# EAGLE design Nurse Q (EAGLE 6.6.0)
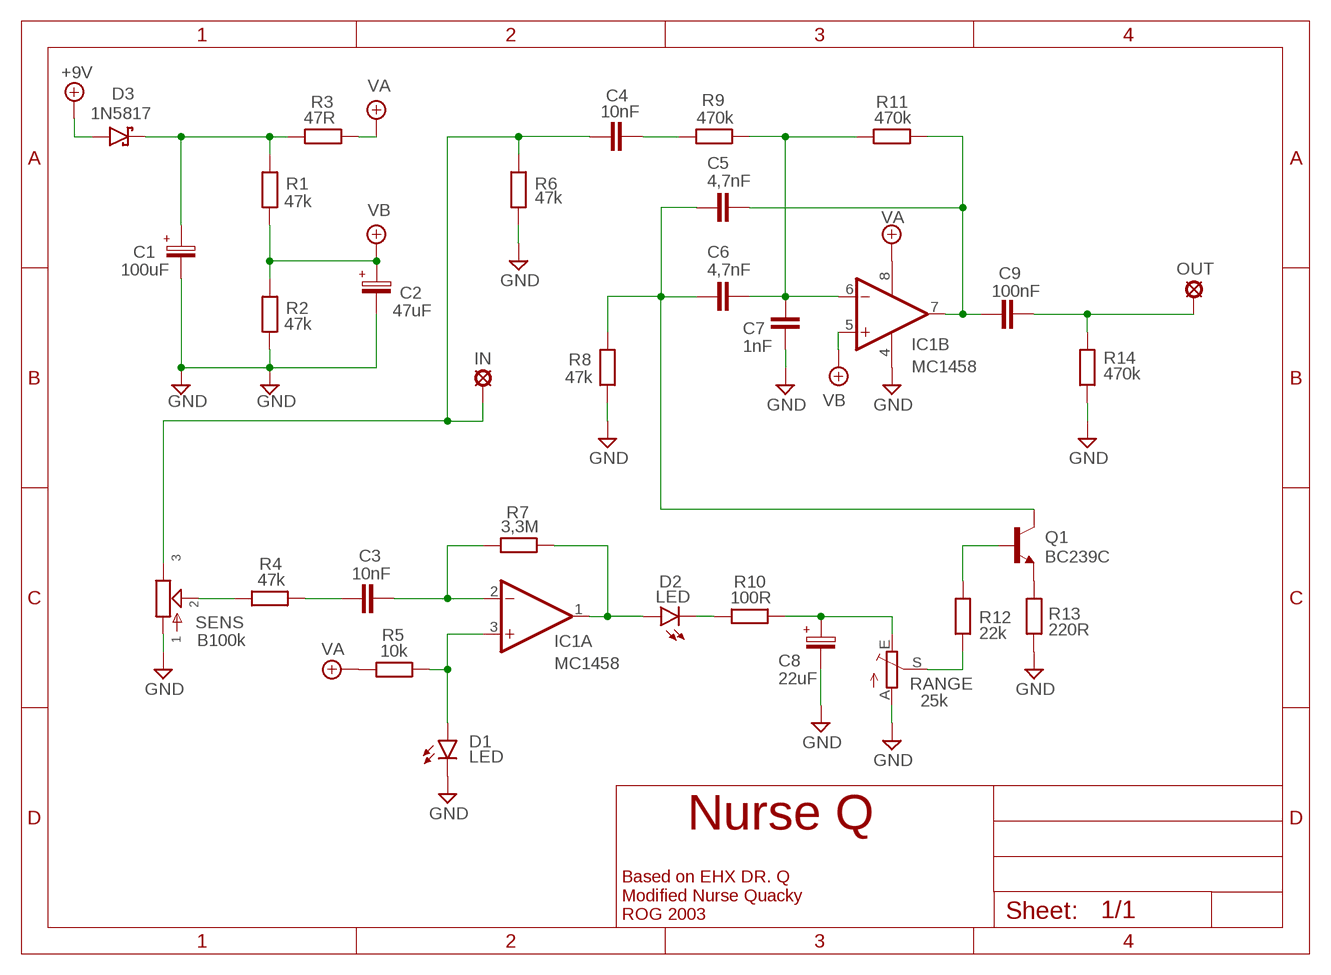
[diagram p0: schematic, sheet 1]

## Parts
+9V  +9V  +9V(T)1  [ROUND]
C1  100uF  063-EU  [063_025]
C2  47uF  063-EU  [063_025]
C3  10nF  1NF-15NF  [3,5MM]
C4  10nF  1NF-15NF  [3,5MM]
C5  4,7nF  1NF-15NF  [3,5MM]
C6  4,7nF  1NF-15NF  [3,5MM]
C7  1nF  1NF-15NF  [3,5MM]
C8  22uF  063-EU  [063_025]
C9  100nF  100NF-220NF  [7,5MM]
D1  LED  LED3MM  [LED3MM]
D2  LED  LED3MM  [LED3MM]
D3  1N5817  [DO41-3]
GND  GND  GND(T)1  [ROUND]
GND1  GND  GND(T)1  [ROUND]
IC1  MC1458  TL072P  [DIL08]
IN  MCS10B  [MCS10B]
OUT  MCS08  [MCS08]
Q1  BC239C  BC5471  [TO92-]
R1  47k  6MM-EU3  [R0207/3]
R2  47k  6MM-EU3  [R0207/3]
R3  47R  6MM-EU3  [R0207/3]
R4  47k  6MM-EU3  [R0207/3]
R5  10k  6MM-EU3  [R0207/3]
R6  47k  6MM-EU3  [R0207/3]
R7  3,3M  6MM-EU3  [R0207/3]
R8  47k  6MM-EU3  [R0207/3]
R9  470k  6MM-EU3  [R0207/3]
R10  100R  6MM-EU3  [R0207/3]
R11  470k  6MM-EU3  [R0207/3]
R12  22k  6MM-EU3  [R0207/3]
R13  220R  6MM-EU3  [R0207/3]
R14  470k  6MM-EU3  [R0207/3]
RANGE  25k  TRIM_EU-PT10  [PT-10]
SENS  B100k  POT-EU16MM  [16MM]

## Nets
+9V: +9V.1(+9V) D3.A
GND: C1.- C2.- C7.1 C8.- D1.K(C) GND1.1(GND) GND.1(GND) IC1.4(P:V-) R2.1 R6.1 R8.1 R13.1 R14.1 RANGE.A SENS.1
N$1: C1.+ D3.C R1.2 R3.1
N$2: C4.1 IN.MP R6.2 SENS.3
N$8: R4.1 SENS.2
N$12: D2.A IC1.1(A:OUT) R7.2
N$18: C6.2 C7.2 IC1.6(B:-IN) R9.2 R11.1
N$19: D2.K(C) R10.1
N$20: C8.+ R10.2 RANGE.E
N$21: R12.1 RANGE.S
N$22: Q1.2(B) R12.2
N$23: Q1.1(E) R13.2
N$24: C4.2 R9.1
N$27: C5.1 C6.1 Q1.3(C) R8.2
N$28: C5.2 C9.P$1 IC1.7(B:OUT) R11.2
N$30: C3.2 IC1.2(A:-IN) R7.1
N$31: C9.P$2 OUT.MP R14.2
N$32: C3.1 R4.2
N$33: D1.A IC1.3(A:+IN) R5.2
VA: IC1.8(P:V+) R3.2 R5.1
VB: C2.+ IC1.5(B:+IN) R1.1 R2.2

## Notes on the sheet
- OUT
- Based on EHX DR. Q
  Modified Nurse Quacky 
  ROG 2003

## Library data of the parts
+9V = gm-supply:+9V(T): +9V Voltage Supply
C1 C2 C8 = Elektrolyytit:063-EU
C3-C7 = Mylar Kondensaattorit:1NF-15NF: 1nF-15nF
C9 = Mylar Kondensaattorit:100NF-220NF: 100nF-220nF
D1 D2 = Diodit:LED
D3 = Diodit:1N5817
GND GND1 = gm-supply:GND(T): Ground
IC1 = Operaatiovahvistimet:TL072: OP AMP
IN = Padit:MCS10B: SOLDER PAD
OUT = solpad:MCS08: SOLDER PAD
Q1 = Transistorit:BC547*: NPN Transistor
R1-R14 = Vastukset:6MM-EU: 6mm Resistors (European schematic symbol)
RANGE = pot:TRIM_EU-: POTENTIOMETER
SENS = gm-pots:POT-EU

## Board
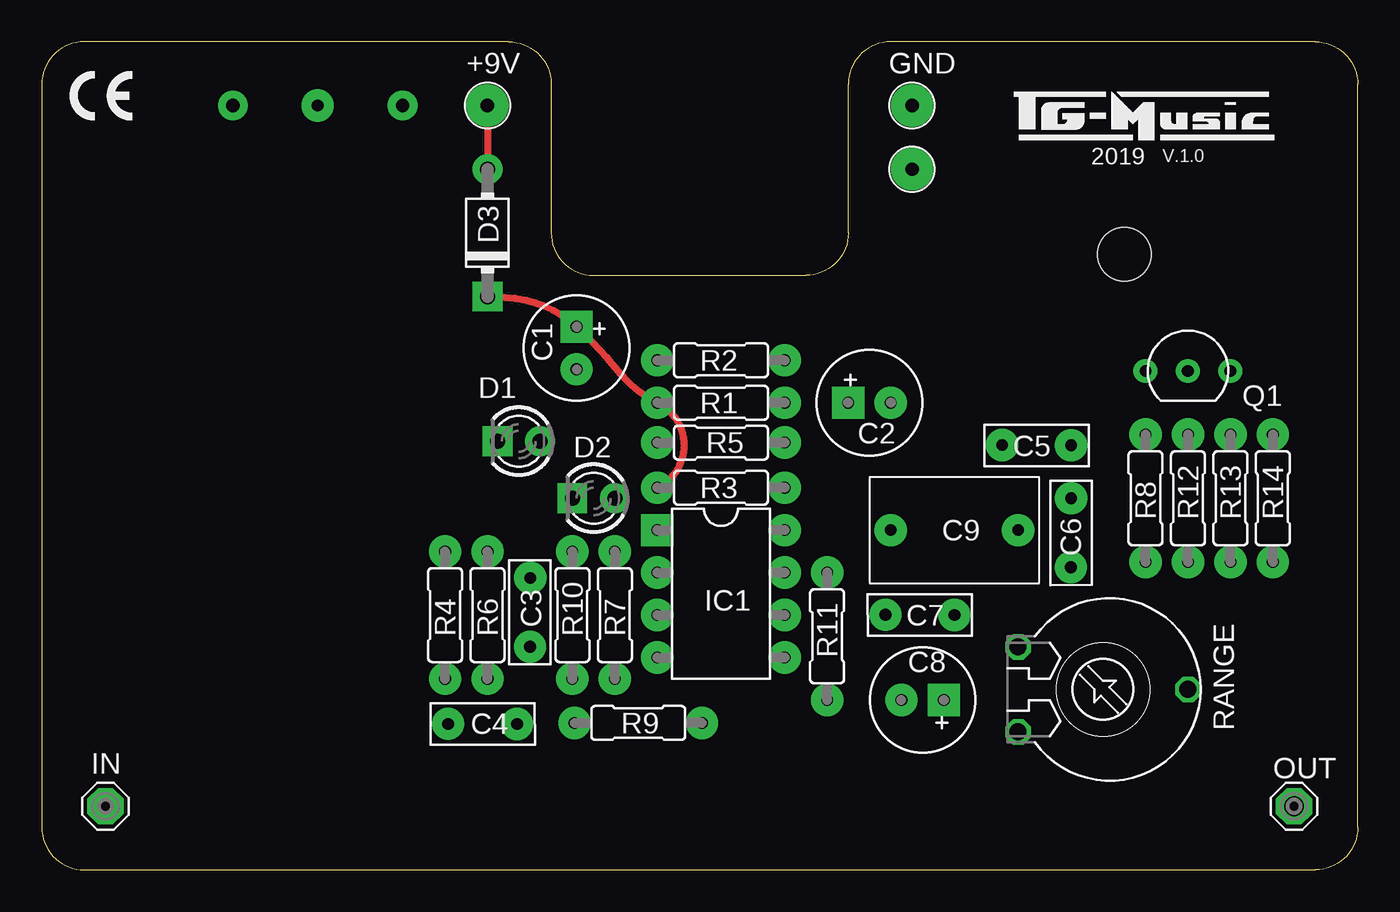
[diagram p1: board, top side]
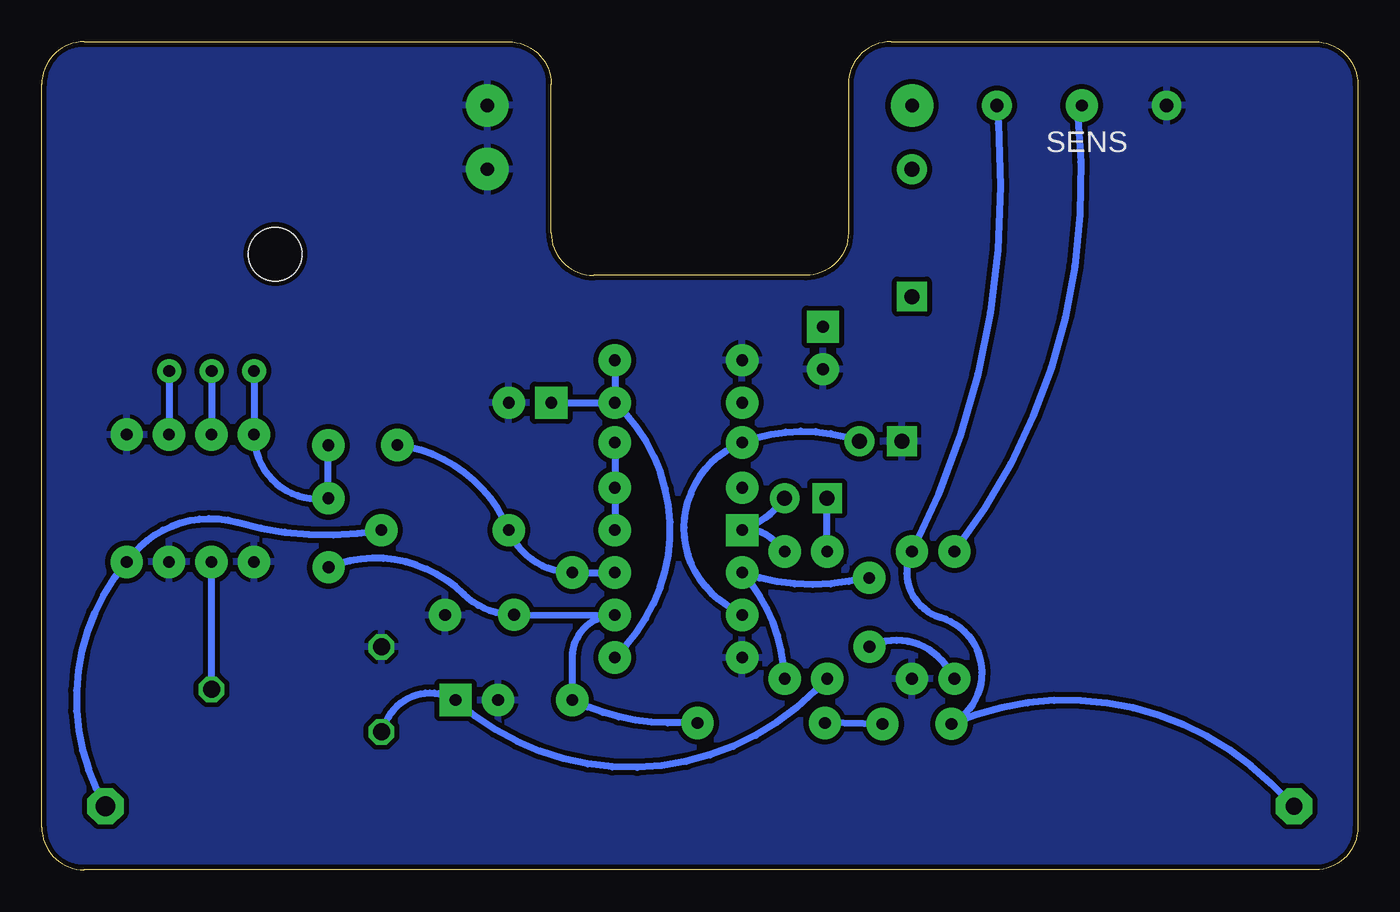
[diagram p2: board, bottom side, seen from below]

Size 78.74 x 49.53 mm. Coordinates in mm from the lower left corner, seen from the top.
Outline: 7.62,49.53 3.81,49.53
Outline: 78.74,2.54 78.74,46.99 arc90 76.2,49.53 50.8,49.53 arc90 48.26,46.99 48.26,38.1 arc-90 45.72,35.56 33.02,35.56 arc-90 30.48,38.1 30.48,46.99 arc90 27.94,49.53 2.54,49.53 arc90 0,46.99 0,2.54 arc90 2.54,0 76.2,0 arc90 78.74,2.54
Copper layers (1*16): Top 0.035mm / dielectric 1.5mm / Bottom 0.035mm
Design rules "ITEADstudio": minimum track width 10mil, minimum drill 12mil, track to track 12mil, track to pad 12mil, pad to pad 12mil, via to via 12mil, smd to smd 0mil, copper to edge 12mil, drill to drill 12mil, minimum pad ring 10mil, minimum via ring 6mil, stop-mask expansion 4mil, vias tented up to drill 100mil, thermal gap 10mil
Holes 3.2 mm at 64.77,36.83

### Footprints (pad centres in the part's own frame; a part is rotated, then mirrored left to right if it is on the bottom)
ROUND = drill 0.8 pad 2.54: 1 0,0
063_025 = drill 0.7 pad 1.93 square: + -1.27,0 | drill 0.7 pad 1.93: - 1.27,0
3,5MM = drill 0.7 pad 1.93: 1 -1.905,0; 2 2.221,-0.016
7,5MM = drill 0.7 pad 1.93: P$1 -3.81,0; P$2 3.81,0
LED3MM = drill 0.9 pad 1.778: A -1.27,0 | drill 0.9 pad 1.778 square: K 1.27,0
DO41-3 = drill 0.9 pad 1.778: A 3.81,0 | drill 0.9 pad 1.778 square: C -3.81,0
DIL08 = drill 0.7 pad 1.93 square: 1 -3.81,-3.81 | drill 0.7 pad 1.93: 2 -1.27,-3.81; 3 1.27,-3.81; 4 3.81,-3.81; 5 3.81,3.81; 6 1.27,3.81; 7 -1.27,3.81; 8 -3.81,3.81
MCS10B = drill 1.016 pad 2.159 octagon: MP 0,0
MCS08 = drill 1.194 pad 2.159 octagon: MP 0,0
TO92- = drill 0.7 pad 1.422: 1 2.54,0; 2 0,0; 3 -2.54,0
R0207/3 = drill 0.7 pad 1.93: 1 -3.81,0; 2 3.81,0
PT-10 = drill 1.016 octagon: A -2.54,-5.08; E 2.54,-5.08; S 0,5.08
16MM = drill 0.8 pad 1.778: 1 5.08,0; 3 -5.08,0 | drill 0.7 pad 1.93: 2 0,0

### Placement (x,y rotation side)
+9V  26.67,45.72 0 top
C1  32,31.21 270 top
C2  49.53,27.94 0 top
C3  29.21,15.24 90 top
C4  26.22,8.73 0 top
C5  59.69,25.4 180 top
C6  61.6,20.32 270 top
C7  52.71,15.24 180 top
C8  52.7,10.16 180 top
C9  54.61,20.32 0 top
D1  28.54,25.63 180 top
D2  33.02,22.23 180 top
D3  26.67,38.1 90 top
GND  52.07,45.72 0 top
GND1  52.07,41.91 0 top
IC1  40.64,16.51 270 top
IN  3.81,3.81 0 top
OUT  74.93,3.81 0 top
Q1  68.58,29.84 0 top
R1  40.64,27.94 180 top
R2  40.64,30.48 0 top
R3  40.64,22.86 0 top
R4  24.13,15.24 270 top
R5  40.64,25.56 180 top
R6  26.67,15.24 90 top
R7  34.29,15.24 90 top
R8  66.04,22.23 90 top
R9  35.69,8.79 0 top
R10  31.75,15.24 270 top
R11  46.99,13.97 90 top
R12  68.58,22.23 90 top
R13  71.12,22.23 90 top
R14  73.66,22.23 270 top
RANGE  63.5,10.79 270 top
SENS  16.51,45.72 0 bottom

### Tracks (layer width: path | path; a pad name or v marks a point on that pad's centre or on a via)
+9V
  Top 0.406: +9V.1 D3.A
GND
  pour Bottom: 0,2.54 0,46.99 arc-90 2.54,49.53 27.94,49.53 arc-90 30.48,46.99 30.48,38.1 arc90 33.02,35.56 45.72,35.56 arc90 48.26,38.1 48.26,46.99 arc-90 50.8,49.53 76.2,49.53 arc-90 78.74,46.99 78.74,2.54 arc-90 76.2,0 2.54,0 arc-90
N$1
  Top 0.406: D3.C 27.71,34.25 arc-40 C1.+ arc-8 34.66,29.65 arc25 R1.2 arc-128 R3.1
N$2
  Bottom 0.406: SENS.3 21.51,44.65 arc32 R6.2 arc-101 24.98,15.11 arc135 C4.1 arc67 5.21,5.18 IN.MP
N$8
  Bottom 0.406: R4.1 arc-44 16.78,45.45 SENS.2
N$12
  Bottom 0.406: D2.A arc28 36.19,20.63 IC1.1 arc53 34.92,19.68 R7.2
N$18
  Bottom 0.406: C6.2 arc66 53.49,16.49 arc-44 C7.2 IC1.6 arc-90 46.99,12.7 R11.1 arc-26 41.27,8.8 R9.2
N$19
  Bottom 0.406: R10.1 D2.K
N$20
  Bottom 0.406: RANGE.E 58.11,8.92 arc97 C8.+ arc-87 32.47,10.7 R10.2
N$21
  Bottom 0.406: RANGE.S R12.1
N$22
  Bottom 0.406: Q1.2 R12.2
N$23
  Bottom 0.406: Q1.1 R13.2
N$24
  Bottom 0.406: C4.2 R9.1
N$27
  Bottom 0.406: C5.1 C6.1 arc99 R8.2 Q1.3
N$28
  Bottom 0.406: C5.2 arc60 C9.P$1 arc-67 R11.2 IC1.7
N$30
  Bottom 0.406: R7.1 arc-40 IC1.2 arc-29 30.45,17.25 C3.2
N$31
  Bottom 0.406: C9.P$2 arc26 67.03,20.79 arc-66 73.25,18.9 R14.2 arc-71 OUT.MP
N$32
  Bottom 0.406: R4.2 24.5,12.02 arc-84 C3.1
N$33
  Bottom 0.406: IC1.3 37.81,15.87 arc126 R5.2 arc41 D1.A
VA
  Bottom 0.406: R5.1 R3.2 IC1.8
VB
  Bottom 0.406: C2.+ 44.5,27.94 R1.1 | R2.2 R1.1 | IC1.5 43.8,13.43 arc-89 R1.1

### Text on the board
tNames: 2019 | V.1.0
